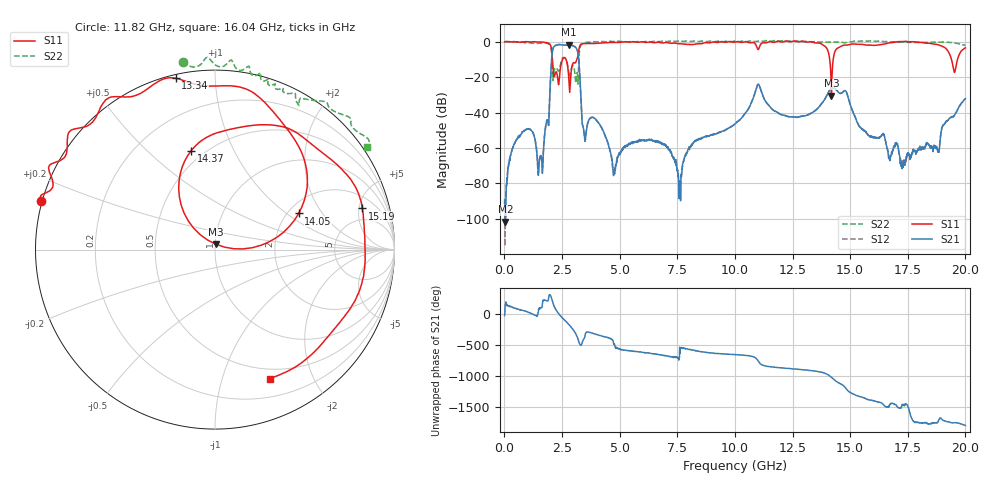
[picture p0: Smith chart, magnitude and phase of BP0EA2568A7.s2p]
! 9/17/2020 12:40:54 PM
! C:\ANRITSUVNA\DATA\MLO\SAMPLES\RAYTHEOM BP\17362_20GH_91720 .S2P
! CHANNEL.1
! TR.MEASUREMENT
! CORRECTED.DATA
# GHZ S RI R 50.0
! FREQ.GHZ  S11RE  S11IM  S31RE  S31IM  S13RE  S13IM  S33RE  S33IM
!; PortSelection: Port_13
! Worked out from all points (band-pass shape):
!   1601 points, 10 MHz to 20 GHz, reference 50 ohm
!   highest |S21| = -1.69 dB at 2.796 GHz (marker M1); lowest = -101.5 dB at 47.48 MHz (marker M2)
!   |S21| within 3 dB of the highest: 2.095 GHz to 3.156 GHz (1.061 GHz wide, 40.4 % of centre)
!   lowest |S11| = -30.4 dB at 14.19 GHz (marker M3), VSWR 1.06, Z = 50.4 + j2.99 ohm
!   |S11| at or under -10 dB: 2.084 GHz to 2.527 GHz (442.4 MHz wide, 19.2 % of centre); 2.672 GHz to 3.145 GHz (473.3 MHz wide, 16.3 % of centre); 19.39 GHz to 19.66 GHz (265.3 MHz wide, 1.36 % of centre)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
!   |S22| runs from -24.0 to 0.6 dB; largest |S21 - S12| = 0.0069
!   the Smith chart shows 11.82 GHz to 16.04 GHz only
!   S11 on the Smith chart (normalised r, x): 11.82 GHz: -0.00, +0.14; 13.34 GHz: 0.02, +0.80; 14.05 GHz: 2.28, +1.24; 14.37 GHz: 0.43, +0.70; 15.19 GHz: 3.23, +5.41; 16.04 GHz: 0.39, -1.44
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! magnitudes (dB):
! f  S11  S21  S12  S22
! 10 MHz  -0.2  -91.2  -88.4  0.0
! 47.48 MHz  0.0  -101.5  -89.7  -0.1
! 934.5 MHz  0.0  -49.6  -49.5  -0.6
! 1.572 GHz  -0.2  -64.6  -64.2  -0.9
! 2.134 GHz  -18.4  -3.2  -3.1  -18.3
! 2.796 GHz  -20.9  -1.7  -1.7  -18.1
! 3.146 GHz  -10.0  -4.4  -4.4  -17.8
! 3.346 GHz  -1.4  -38.9  -38.8  -1.7
! 4.758 GHz  -0.5  -72.9  -73.9  0.0
! 6.682 GHz  -0.4  -56.1  -55.9  0.0
! 7.594 GHz  -1.3  -85.5  -81.1  0.3
! 10.01 GHz  -0.3  -46.3  -46.3  0.2
! 11 GHz  -4.5  -24.1  -24.1  0.3
! 11.82 GHz  0.0  -39.7  -39.7  0.5
! 13.34 GHz  -0.2  -40.1  -40.1  -0.2
! 14.05 GHz  -5.9  -28.7  -28.6  -0.4
! 14.19 GHz  -30.4  -26.3  -26.3  -0.2
! 14.37 GHz  -4.9  -26.9  -26.8  -0.4
! 15.19 GHz  -1.4  -41.7  -41.8  0.2
! 16.04 GHz  -2.2  -54.1  -54.2  0.2
! 16.68 GHz  -0.7  -64.9  -65.3  0.0
! 20 GHz  -3.5  -32.2  -32.2  -2.1
